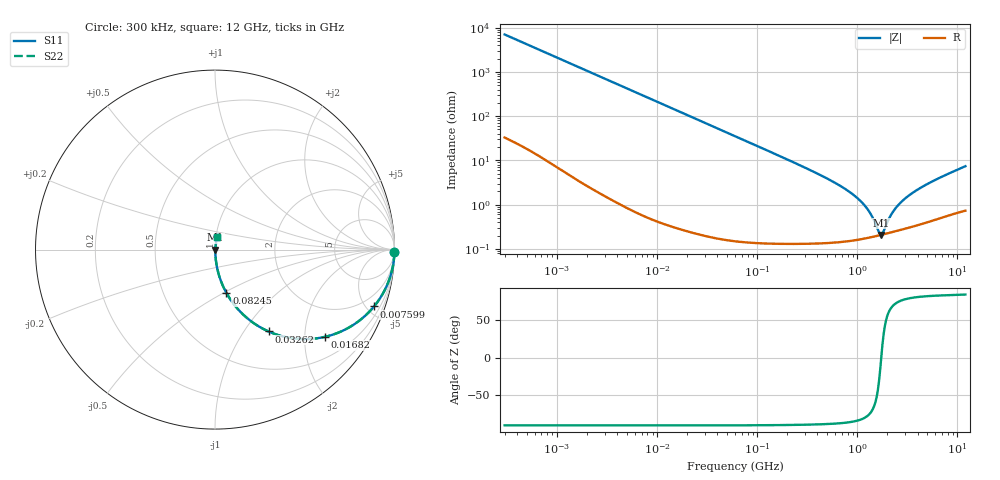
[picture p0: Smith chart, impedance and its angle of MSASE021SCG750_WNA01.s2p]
! MSASE021SCG750_WNA01  S-PARAMETER MODEL  ( Standard Model )
! Model Generated by TAIYO YUDEN Corporation (http://www.ty-top.com)
! Version 1.0
! TAIYO YUDEN Control No. 241126
! Copyright(c) 2024 TAIYO YUDEN CO.,LTD. All Rights Reserved.
! Product Description (link to TY-COMPAS)
! https://ds.yuden.co.jp/TYCOMPAS/or/detail?pn=MSASE021SCG750GWNA01&u=M
! Products Name : Multilayer Ceramic Capacitors
! Characteristics :
!  Capacitance : 75 [pF] , Rated Voltage : 16 [V] , TCC : CG / C0G
!  Case Size : 0.25 x 0.125 / 0.0098 x 0.0049 [mm/inch] , Thickness : 0.125 / 0.0049 [mm/inch]
!  (Conditions: Temperature = 25 [degC] , DC Bias Voltage = 0 [V])
! External Node Assignments :
!  1  o---| |---o  2
! GND o---------o GND
! Frequency Range : 0.3MHz  -  12000MHz  [ 401 STEP ]
# MHZ S RI R 50
! Freq[MHz].  S11 Real  S11 Imag  S21 Real  S21 Imag  S12 Real  S12 Imag  S22 Real  S22 Imag
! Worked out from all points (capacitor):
!   401 points, 300 kHz to 12 GHz, reference 50 ohm
!   read as one part in series: C = 75.4 pF near 316.3 kHz
!   lowest |Z| = 208 mohm at 1.735 GHz (marker M1)
!   series resonance near 1.732 GHz, so ESL is about 110 pH
!   S11 on the Smith chart (normalised r, x): 300 kHz: open; 7.599 MHz: 1.01, -5.59; 16.82 MHz: 1.01, -2.52; 32.62 MHz: 1.00, -1.30; 82.45 MHz: 1.00, -0.51; 12 GHz: 1.01, +0.15
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0.3  0.9997 -0.0142  0.000269 0.0142  0.000269 0.0142  0.9997 -0.0142
1.769972  0.9929 -0.0829  0.00714 0.0829  0.00714 0.0829  0.9929 -0.0829
4.242641  0.9612 -0.1922  0.0388 0.1922  0.0388 0.1922  0.9612 -0.1922
7.598879  0.8859 -0.317  0.1141 0.317  0.1141 0.317  0.8859 -0.317
10.44266  0.8047 -0.3955  0.1953 0.3955  0.1953 0.3955  0.8047 -0.3955
16.82302  0.6142 -0.4857  0.3858 0.4857  0.3858 0.4857  0.6142 -0.4857
32.62367  0.2982 -0.456  0.7018 0.456  0.7018 0.456  0.2982 -0.456
60  0.1123 -0.3136  0.8877 0.3136  0.8877 0.3136  0.1123 -0.3136
82.45425  0.0632 -0.2406  0.9368 0.2406  0.9368 0.2406  0.0632 -0.2406
159.8975  0.0183 -0.1292  0.9817 0.1292  0.9817 0.1292  0.0183 -0.1292
353.9943  0.00459 -0.0571  0.9954 0.0571  0.9954 0.0571  0.00459 -0.0571
668.5285  0.00214 -0.0268  0.9979 0.0268  0.9979 0.0268  0.00214 -0.0268
1021.415  0.00179 -0.0134  0.9982 0.0134  0.9982 0.0134  0.00179 -0.0134
1296.429  0.00183 -0.00705  0.9982 0.00705  0.9982 0.00705  0.00183 -0.00705
1645.489  0.00201 -0.00122  0.998 0.00122  0.998 0.00122  0.00201 -0.00122
1735.023  0.00207 4.48e-05  0.9979 -4.48e-05  0.9979 -4.48e-05  0.00207 4.48e-05
1829.429  0.00214 0.0013  0.9979 -0.0013  0.9979 -0.0013  0.00214 0.0013
2088.533  0.00232 0.00444  0.9977 -0.00444  0.9977 -0.00444  0.00232 0.00444
2581.562  0.0027 0.00958  0.9973 -0.00958  0.9973 -0.00958  0.0027 0.00958
3642.919  0.00357 0.0187  0.9964 -0.0187  0.9964 -0.0187  0.00357 0.0187
6026.253  0.00582 0.0357  0.9942 -0.0357  0.9942 -0.0357  0.00582 0.0357
12000  0.0125 0.0721  0.9875 -0.0721  0.9875 -0.0721  0.0125 0.0721
